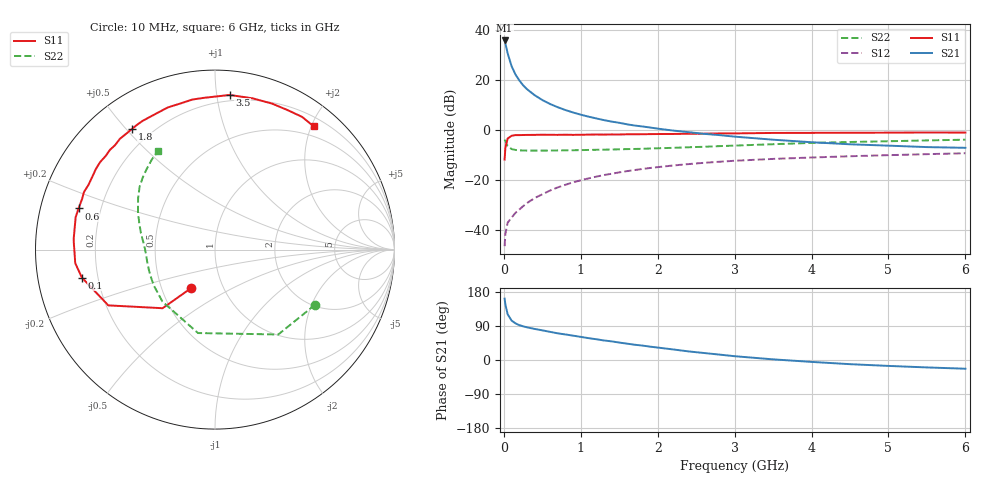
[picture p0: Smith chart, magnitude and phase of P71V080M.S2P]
! SIEMENS Small Signal Semiconductors
! BFP196
! Si NPN RF Bipolar Junction Transistor in SOT143
! VCE = 1 V  IC = 80 mA
! Common Emitter S-Parameters:  May  1996
# GHz  S  MA  R  50
!  f  S11  S21  S12  S22
! GHz  MAG  ANG  MAG  ANG  MAG  ANG  MAG  ANG
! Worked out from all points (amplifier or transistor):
!   36 points, 10 MHz to 6 GHz, reference 50 ohm
!   highest |S21| = 35.7 dB at 10 MHz (marker M1)
!   |S21| within 3 dB of that: start of sweep to 33.64 MHz
!   unconditionally stable (mu >= 1): 230.5 MHz to end of sweep
!   at 250 MHz: K = 1.02, MAG = 23.3 dB, |S12| = -30.6 dB
!   at 1.4 GHz: K = 1.15, MAG = 8.1 dB, |S12| = -17.6 dB
!   at 6 GHz: K = 1.05, MAG = -0.3 dB, |S12| = -9.4 dB
!   S11 on the Smith chart (normalised r, x): 10 MHz: 0.70, -0.32; 100 MHz: 0.14, -0.10; 600 MHz: 0.12, +0.15; 1.8 GHz: 0.13, +0.52; 3.5 GHz: 0.16, +1.09; 6 GHz: 0.34, +2.04
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0.01  0.2535 -121.9  61.29 161.9  0.0047 69.6  0.637 -28.8
0.02  0.4381 -131.8  53.49 146.3  0.0083 62.4  0.59 -53.3
0.05  0.6707 -152.4  33.75 120.5  0.0139 47.5  0.4744 -101.5
0.1  0.7579 -168.1  18.86 104.2  0.0175 46.1  0.412 -135.3
0.15  0.7825 -174.5  12.9 96.8  0.0217 51.8  0.3952 -149.7
0.2  0.7828 -178.9  9.775 92.1  0.0253 56.2  0.3884 -157.3
0.25  0.7867 177.8  7.789 88.9  0.0296 58.7  0.3857 -162.5
0.3  0.7897 175.5  6.517 86.3  0.0341 61.6  0.3841 -165.7
0.4  0.7918 170.4  4.927 82.0  0.0431 63.8  0.3838 -170.4
0.5  0.7971 167.0  3.945 78.3  0.0512 64.9  0.384 -173.5
0.6  0.7941 163.2  3.29 74.3  0.0609 65.3  0.3847 -175.6
0.7  0.7923 159.2  2.832 70.4  0.0703 64.9  0.3865 -177.5
0.8  0.7973 156.3  2.487 67.4  0.0795 63.9  0.3888 -179.2
1.1  0.8012 146.1  1.834 57.7  0.1066 60.7  0.3954 176.8
1.4  0.807 136.5  1.461 49.2  0.132 56.1  0.4034 173.3
1.8  0.8162 124.4  1.167 38.1  0.1645 49.8  0.4166 168.6
2.2  0.8251 113.9  0.966 27.9  0.1932 43.2  0.4356 163.6
3  0.8476 94.4  0.73 10.0  0.2401 30.4  0.4829 152.7
3.5  0.8654 84.6  0.634 1.7  0.2617 23.2  0.515 146.3
4.5  0.8733 68.7  0.513 -11.0  0.296 10.9  0.5703 134.7
5.5  0.8844 56.7  0.451 -19.6  0.3258 0.1  0.6136 124.9
6  0.8796 51.3  0.436 -23.0  0.3399 -5.8  0.634 120.0
